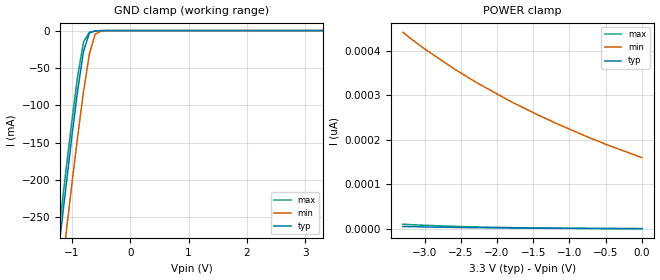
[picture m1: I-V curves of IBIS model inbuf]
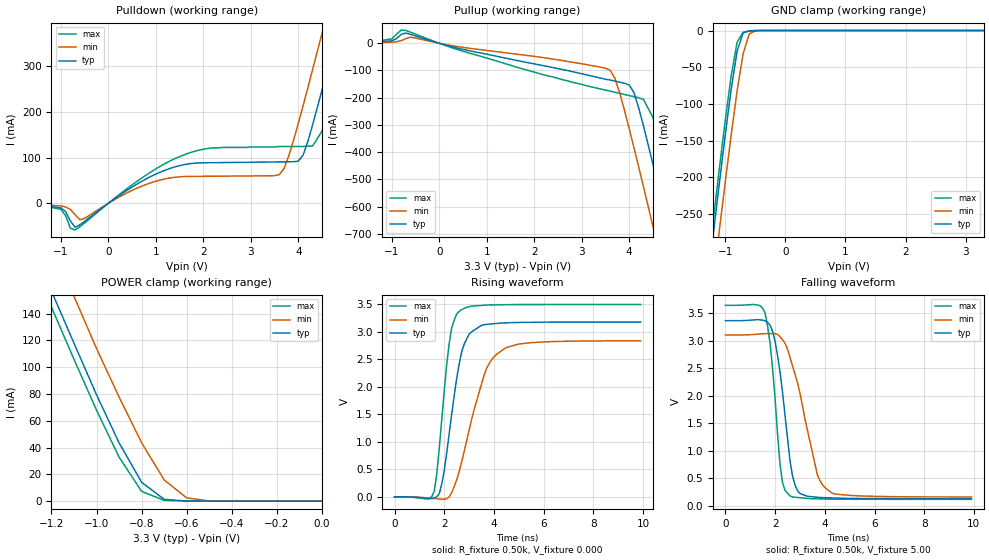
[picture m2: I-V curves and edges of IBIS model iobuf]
| IBIS file 63245l.ibs created by s2ibis2 version 1.0
| North Carolina State University Electronics Research Laboratory  1995
[IBIS ver]   2.1
[File name]   63245l.ibs
[File Rev]   0.1
[Date]   Friday, August 15, 1997
[Source]   IDT
[Notes]   1. Temp typ=25C, min=100C, max=0C 2. Ramp rates based on 500
   ohm load
[Copyright]   Copyright 1997, Integrated Device Technology, Inc.
[Disclaimer] Integrated Device Technology, Inc. ("IDT") hereby grants the
   user of this IBIS model a non-exclusive, nontransferable
   license to use this IBIS model under the following terms.
   The user is granted this license only to use the IBIS model
   and is not granted rights to sell, copy (except as needed to
   run the IBIS model), rent, lease or sub-license the IBIS model
   in whole or in part, or in modified form to anyone.
   The User may modify the IBIS model to suit its specific
   applications, but rights to derivative works and such
   modifications shall belong to IDT.
   This IBIS model is provided on an "AS IS" basis and IDT
   makes absolutely no warranty with respect to the information
   contained herein. IDT DISCLAIMS AND CUSTOMER WAIVES ALL
   WARRANTIES, EXPRESS AND IMPLIED, INCLUDING WARRANTIES OF
   MERCHANTABILITY AND FITNESS FOR A PARTICULAR PURPOSE. THE
   ENTIRE RISK AS TO QUALITY AND PERFORMANCE IS WITH THE
   USER ACCORDINGLY, IN NO EVENT SHALL IDT BE LIABLE
   FOR ANY DIRECT OR INDIRECT DAMAGES, WHETHER IN CONTRACT OR
   TORT, INCLUDING ANY LOST PROFITS OR OTHER INCIDENTAL,
   CONSEQUENTIAL, EXEMPLARY, OR PUNITIVE DAMAGES ARISING OUT OF
   THE USE OR APPLICATION OF THE IBIS model.  Further, IDT
   reserves the right to make changes without notice to any
   product herein to improve reliability, function, or design.
   IDT does not convey any license under patent rights or
   any other intellectual property rights, including those of
   third parties. IDT is not obligated to provide maintenance
   or support for the licensed IBIS model.
|   Component IDT54/74FCT163245/A/C
[Component]   IDT54/74FCT163245/A/C
[Manufacturer]   Integrated Device Technology Inc.
[Package]
| Following package parameters are for SO48-2(TSSOP) package
|[Package]
|| variable   typ   min   max
|R_pkg   15.00m   10.00m   20.00m
|L_pkg   2.30nh   1.40nh   4.50nH
|C_pkg   0.40pF   0.35pF   0.60pF
| Following package parameters are for SO48-1(SSOP), E48-1(CERPAK) packages
| variable   typ   min   max
R_pkg   15.00m   10.00m   20.00m
L_pkg   2.90nH   1.50nH   5.60nH
C_pkg   0.40pF   0.26pF   0.50pF
[Pin]  signal_name   model_name   R_pin   L_pin   C_pin
1   1DIR   inbuf
2   1B1   iobuf
3   1B2   iobuf
4   GND   GND
5   1B3   iobuf
6   1B4   iobuf
7   VCC   POWER
8   1B5   iobuf
9   1B6   iobuf
10   GND   GND
11   1B7   iobuf
12   1B8   iobuf
13   2B1   iobuf
14   2B2   iobuf
15   GND   GND
16   2B3   iobuf
17   2B4   iobuf
18   VCC   POWER
19   2B5   iobuf
20   2B6   iobuf
21   GND   GND
22   2B7   iobuf
23   2B8   iobuf
24   2DIR   inbuf
25   2OEB   inbuf
26   2A8   iobuf
27   2A7   iobuf
28   GND   GND
29   2A6   iobuf
30   2A5   iobuf
31   VCC   POWER
32   2A4   iobuf
33   2A3   iobuf
34   GND   GND
35   2A2   iobuf
36   2A1   iobuf
37   1A8   iobuf
38   1A7   iobuf
39   GND   GND
40   1A6   iobuf
41   1A5   iobuf
42   VCC   POWER
43   1A4   iobuf
44   1A3   iobuf
45   GND   GND
46   1A2   iobuf
47   1A1   iobuf
48   1OEB   inbuf
| Models and submodels in the file (2): inbuf (Input), iobuf (I/O)
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| in   IN1   dummy_model
| oe   OE1   dummy_model
|   Model inbuf
[Model]   inbuf
Model_type   Input
Vinl =  0.800V
Vinh =  2.000V
C_comp   3.00pF   NA   NA
[Temperature Range]   25.00   100.00   0.000
[Voltage Range]   3.30V   3.00V   3.60V
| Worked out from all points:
|   GND clamp passes 1 mA (typ) near -0.62 V on its own axis
[GND_clamp]
| voltage   I(typ)   I(min)   I(max)
-3.3V     -1.781A    -1.841A    -1.762A
-1.3V     -346mA     -410mA     -324mA
-1.2V     -276mA     -341mA     -255mA
-1.1V     -209mA     -273mA     -187mA
-1V       -142mA     -206mA     -122mA
-900mV    -80.26mA   -142mA     -61.07mA
-800mV    -27.87mA   -81.82mA   -15.26mA
-700mV    -3.289mA   -31.47mA   -2.24mA
-600mV    -480uA     -4.848mA   -551uA
-500mV    -82.77uA   -464uA     -85.69uA
3.3V      588fA      178pA      482fA
[POWER_clamp]
| voltage   I(typ)   I(min)   I(max)
-3.3V     5.432pA    441pA      10.51pA
-3V       4.444pA    404pA      8.155pA
-2.6V     3.398pA    360pA      5.808pA
-2.3V     2.779pA    330pA      4.5pA
-1.8V     1.984pA    285pA      2.938pA
-1.2V     1.325pA    238pA      1.756pA
-700mV    945fA      203pA      1.142pA
0V        588fA      160pA      625fA
|   Model iobuf
[Model]   iobuf
Model_type   I/O
Polarity   Non-Inverting
Enable   Active-High
Vinl =  0.800V
Vinh =  2.000V
C_comp   3.00pF   NA   NA
[Temperature Range]   25.00   100.00   0.000
[Voltage Range]   3.30V   3.00V   3.60V
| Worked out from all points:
|   slope of the pulldown table from 0 to 0.495 V, typ, clamps not added: 14.1 ohm
|   slope of the pullup table from 0 to 0.495 V, typ, clamps not added: 22.2 ohm
|   GND clamp passes 1 mA (typ) near -0.62 V on its own axis
|   POWER clamp passes 1 mA (typ) near -0.67 V on its own axis
|   rising waveform, R_fixture 0.50k, V_fixture 0.000: 20-80 % time 609ps typ, 986ps min, 442ps max; typ from 0 V to 3.17 V
|   falling waveform, R_fixture 0.50k, V_fixture 5.00: 20-80 % time 512ps typ, 891ps min, 384ps max; typ from 3.36 V to 0.129 V
[Pulldown]
| voltage   I(typ)   I(min)   I(max)
-3.3V     -1mA       0A         -1mA
-1V       -10.1mA    -5.8mA     -13.1mA
-700mV    -52.41mA   -25.02mA   -58.28mA
1.5V      82.23mA    57.84mA    102mA
3.6V      90.38mA    62.61mA    124mA
3.8V      90.63mA    104mA      124mA
4.1V      105mA      213mA      124mA
4.3V      171mA      292mA      125mA
4.5V      248mA      372mA      158mA
4.9V      411mA      535mA      311mA
5.1V      494mA      618mA      393mA
6.6V      1.122A     1.24A      1.022A
[Pullup]
| voltage   I(typ)   I(min)   I(max)
-3.3V     0A         1mA        1mA
-1.5V     2.3mA      1.4mA      3mA
-700mV    37.47mA    17.46mA    46.94mA
3.5V      -132mA     -91.52mA   -172mA
3.7V      -139mA     -129mA     -180mA
4.1V      -181mA     -383mA     -196mA
4.3V      -303mA     -526mA     -206mA
4.5V      -444mA     -672mA     -272mA
4.7V      -590mA     -820mA     -406mA
4.9V      -738mA     -968mA     -551mA
5.1V      -887mA     -1.116A    -698mA
6.6V      -2.019A    -2.242A    -1.829A
[GND_clamp]
| voltage   I(typ)   I(min)   I(max)
-3.3V     -1.845A    -1.891A    -1.839A
-1.3V     -351mA     -414mA     -332mA
-1.2V     -280mA     -344mA     -261mA
-1.1V     -211mA     -275mA     -191mA
-1V       -144mA     -208mA     -124mA
-900mV    -80.93mA   -143mA     -62.38mA
-800mV    -28.09mA   -82.05mA   -15.75mA
-700mV    -3.331mA   -31.56mA   -2.343mA
-600mV    -482uA     -4.864mA   -563uA
-500mV    -82.6uA    -465uA     -86.04uA
3.3V      639fA      360nA      501fA
[POWER_clamp]
| voltage   I(typ)   I(min)   I(max)
-3.3V     1.028A     1.052A     1.02A
-1.3V     197mA      231mA      185mA
-1.2V     157mA      192mA      145mA
-1.1V     118mA      153mA      106mA
-1V       79.45mA    114mA      67.95mA
-900mV    43.56mA    77.76mA    32.88mA
-800mV    14.07mA    43.59mA    7.263mA
-700mV    1.334mA    15.8mA     596uA
-600mV    60.43uA    2.386mA    67.13uA
-500mV    2.01uA     169uA      3.696uA
0V        639fA      159pA      682fA
[Ramp]
| variable   typ   min   max
dV/dt_r   1.90/0.61n   1.70/0.99n   2.09/0.44n
dV/dt_f   1.93/0.52n   1.74/0.81n   2.11/0.39n
R_load = 0.50k
[Rising Waveform]
R_fixture = 0.50k
V_fixture = 0.000
| time   V(typ)   V(min)   V(max)
0s        0V         0V         0V
1.6ns     -20.72mV   -29.7mV    106mV
1.9ns     237mV      -42.26mV   1.404V
2.2ns     1.15V      1.166mV    2.789V
2.3ns     1.502V     77.53mV    3.068V
2.6ns     2.412V     456mV      3.365V
3ns       2.955V     1.211V     3.453V
3.7ns     3.13V      2.329V     3.481V
4.4ns     3.156V     2.684V     3.487V
9.9ns     3.172V     2.832V     3.491V
[Falling Waveform]
R_fixture = 0.50k
V_fixture = 5.00
| time   V(typ)   V(min)   V(max)
0s        3.363V     3.103V     3.641V
1.6ns     3.362V     3.126V     3.496V
1.9ns     3.166V     3.129V     2.491V
2.2ns     2.422V     3.072V     746mV
2.3ns     2.059V     3.013V     421mV
2.6ns     817mV      2.695V     179mV
2.9ns     276mV      2.238V     149mV
3.7ns     154mV      564mV      125mV
4.3ns     141mV      227mV      120mV
9.9ns     129mV      158mV      116mV
